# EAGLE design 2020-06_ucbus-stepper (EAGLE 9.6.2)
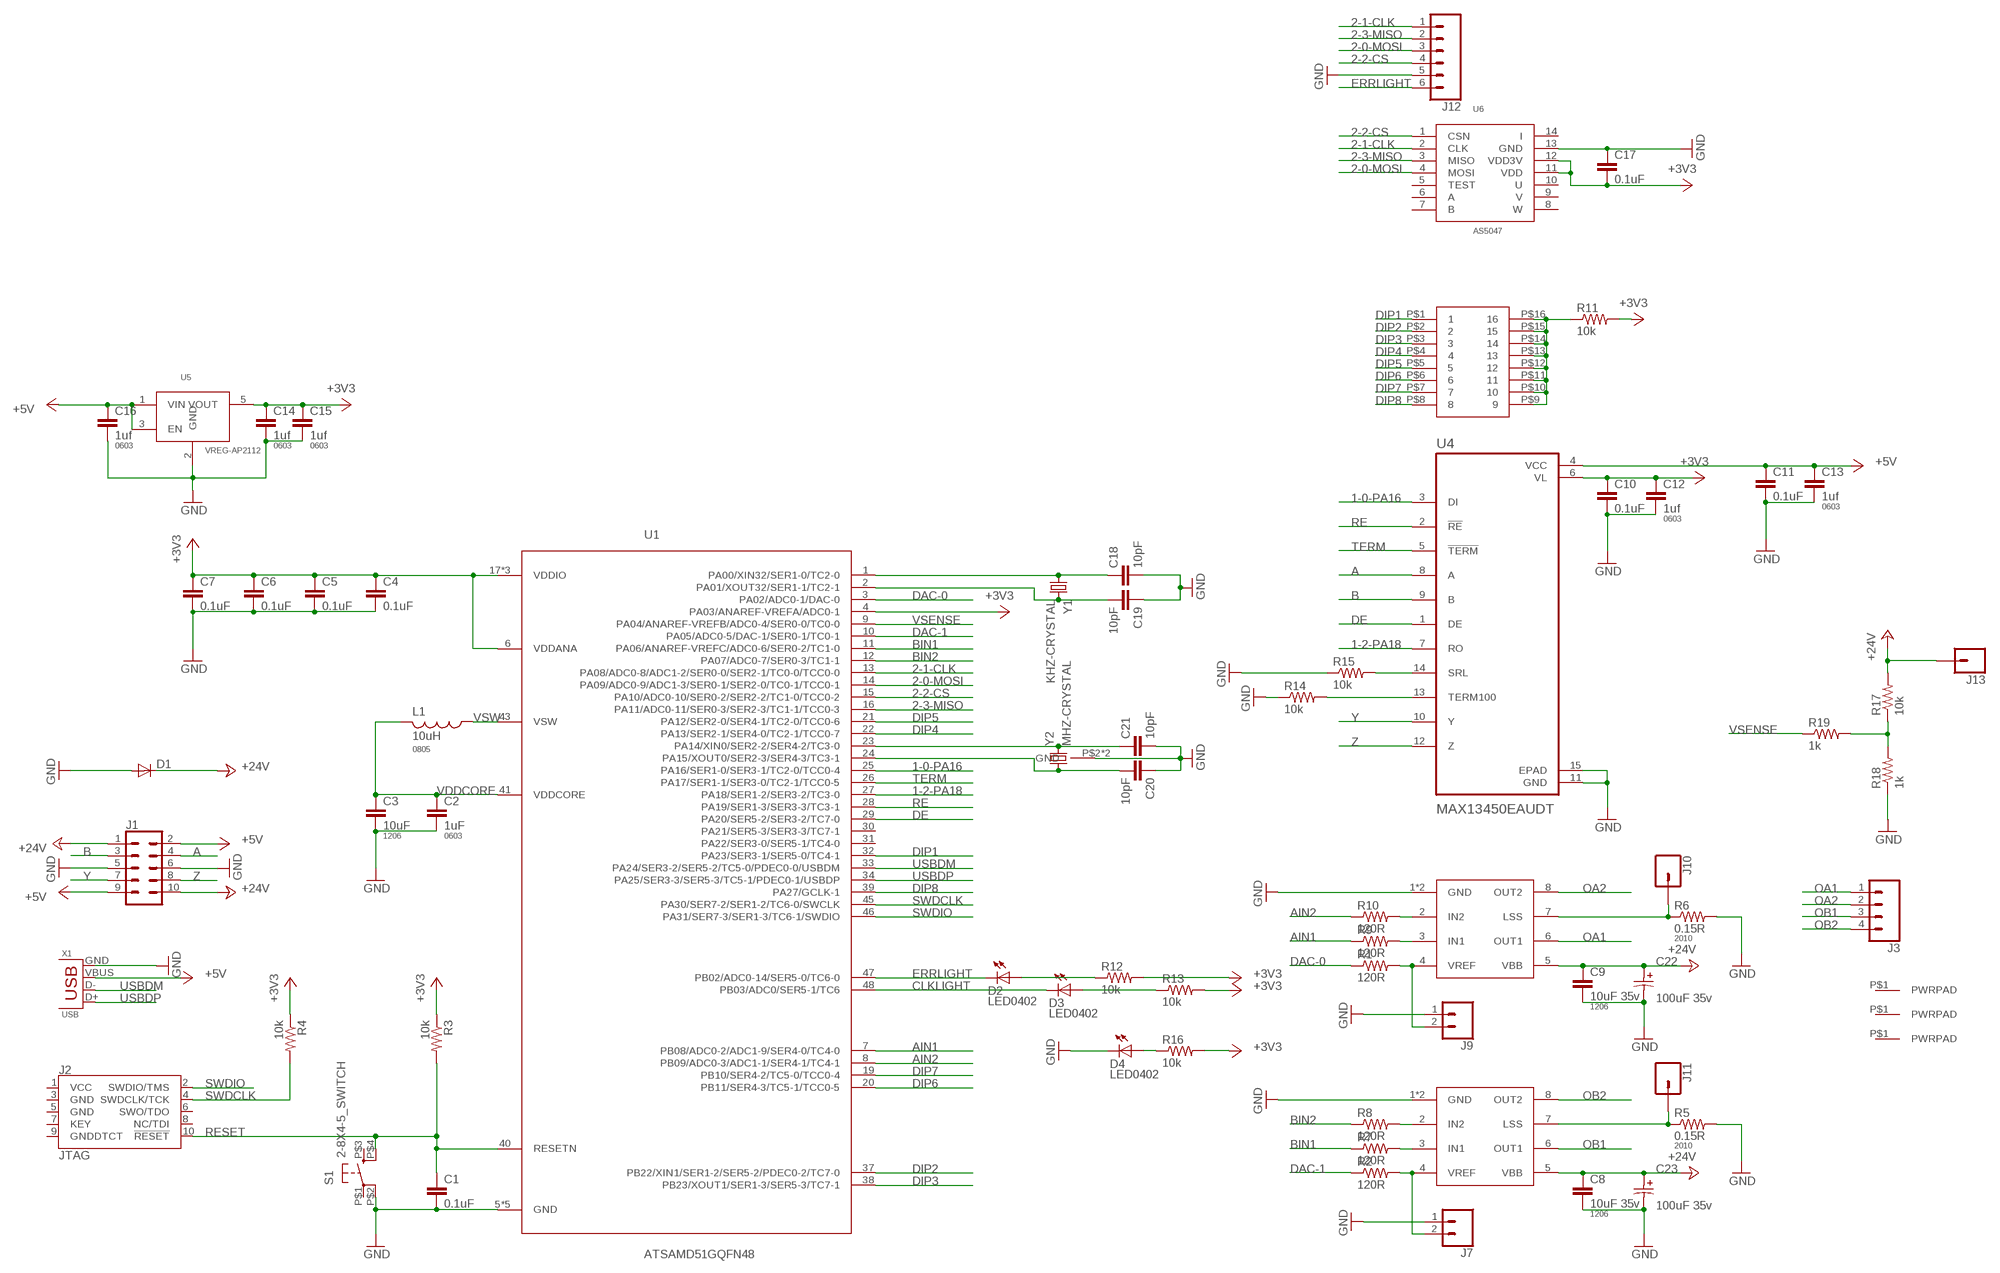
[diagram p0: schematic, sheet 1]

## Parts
C1  0.1uF  CAP0402  [0402]
C2  1uF  CAP0603-CAP  [0603-CAP]
C3  10uF  CAP1206  [1206]
C4  0.1uF  CAP0402  [0402]
C5  0.1uF  CAP0402  [0402]
C6  0.1uF  CAP0402  [0402]
C7  0.1uF  CAP0402  [0402]
C8  10uF 35v  CAP1206  [1206]
C9  10uF 35v  CAP1206  [1206]
C10  0.1uF  CAP0402  [0402]
C11  0.1uF  CAP0402  [0402]
C12  1uf  CAP0603-CAP  [0603-CAP]
C13  1uf  CAP0603-CAP  [0603-CAP]
C14  1uf  CAP0603-CAP  [0603-CAP]
C15  1uf  CAP0603-CAP  [0603-CAP]
C16  1uf  CAP0603-CAP  [0603-CAP]
C17  0.1uF  CAP0402  [0402]
C18  10pF  CAP0402  [0402]
C19  10pF  CAP0402  [0402]
C20  10pF  CAP0402  [0402]
C21  10pF  CAP0402  [0402]
C22  100uF 35v  CAP-POLCAP_POL_SMD6.6X6.6  [SMD-ELEC-CAP]
C23  100uF 35v  CAP-POLCAP_POL_SMD6.6X6.6  [SMD-ELEC-CAP]
D1  DIODESMA403D  [SMA-403D]
D2  LED0402  [0402-D]
D3  LED0402  [0402-D]
D4  LED0402  [0402-D]
J1  CONN_05X2SHD_SMD  [2X5-SHROUDED_SMD]
J2  JTAG  CORTEX_JTAG_DEBUG_SMD  [2X5-SMD-1.27MM]
J3  CONN_04SCREW_LOCK  [SCREWTERMINAL-3.5MM-4_LOCK]
J4  PWRPADM3-SKINNY  [PWRPAD_3-25MM-SKINNY]
J5  PWRPADM3-SKINNY  [PWRPAD_3-25MM-SKINNY]
J6  PWRPADM3-SKINNY  [PWRPAD_3-25MM-SKINNY]
J7  CONN_02LOCK  [1X02_LOCK]
J8  DIPSWITCH-8  [DIPSWITCH-8]
J9  CONN_02LOCK  [1X02_LOCK]
J10  CONN_01PTH_NO_SILK_YES_STOP  [1X01_NO_SILK]
J11  CONN_01PTH_NO_SILK_YES_STOP  [1X01_NO_SILK]
J12  CONN_06SMD-FEMALE-V2  [1X06-SMD-FEMALE]
J13  CONN_01PTH_NO_SILK_YES_STOP  [1X01_NO_SILK]
L1  10uH  INDUCTOR-0805  [0805]
R1  120R  RESISTOR0402  [0402]
R2  120R  RESISTOR0402  [0402]
R3  10k  RESISTOR0402  [0402]
R4  10k  RESISTOR0402  [0402]
R5  0.15R  RESISTOR2010  [R2010]
R6  0.15R  RESISTOR2010  [R2010]
R7  120R  RESISTOR0402  [0402]
R8  120R  RESISTOR0402  [0402]
R9  120R  RESISTOR0402  [0402]
R10  120R  RESISTOR0402  [0402]
R11  10k  RESISTOR0402  [0402]
R12  10k  RESISTOR0402  [0402]
R13  10k  RESISTOR0402  [0402]
R14  10k  RESISTOR0402  [0402]
R15  10k  RESISTOR0402  [0402]
R16  10k  RESISTOR0402  [0402]
R17  10k  RESISTOR0402  [0402]
R18  1k  RESISTOR0402  [0402]
R19  1k  RESISTOR0402  [0402]
S1  2-8X4-5_SWITCH  [TACT-SWITCH-KMR6]
U1  ATSAMD51GQFN48  [QFN-48-7X7MM]
U2  A4950  [SOIC8_PAD]
U3  A4950  [SOIC8_PAD]
U4  MAX13450EAUDT  [SOP65P637X110-14N]
U5  VREG-AP2112  [SOT23-5]
U6  AS5047  [TSSOP14]
X1  USB  [USB_MICRO_609-4613-1-ND]
Y1  KHZ-CRYSTAL  [2-SMD-3.2X1.5MM]
Y2  MHZ-CRYSTAL  [4-SMD-3.2X2.5]

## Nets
1-0-PA16: U1.25(PA16/SER1-0/SER3-1/TC2-0/TCC0-4) U4.3(DI)
1-2-PA18: U1.27(PA18/SER1-2/SER3-2/TC3-0) U4.7(RO)
2-0-MOSI: J12.3 U1.14(PA09/ADC0-9/ADC1-3/SER0-1/SER2-0/TC0-1/TCC0-1) U6.4(MOSI)
2-1-CLK: J12.1 U1.13(PA08/ADC0-8/ADC1-2/SER0-0/SER2-1/TC0-0/TCC0-0) U6.2(CLK)
2-2-CS: J12.4 U1.15(PA10/ADC0-10/SER0-2/SER2-2/TC1-0/TCC0-2) U6.1(CSN)
2-3-MISO: J12.2 U1.16(PA11/ADC0-11/SER0-3/SER2-3/TC1-1/TCC0-3) U6.3(MISO)
+3V3: C4.1 C5.1 C6.1 C7.1 C10.1 C12.1 C14.1 C15.1 C17.2 R3.1 R4.1 R11.2 R12.2 R13.2 R16.2 U1.4(PA03/ANAREF-VREFA/ADC0-1) U1.6(VDDANA) U1.17(VDDIO) U1.36(VDDIO) U1.44(VDDIO) U4.6(VL) U5.5(VOUT) U6.11(VDD) U6.12(VDD3V)
+5V: C11.1 C13.1 C16.1 J1.2 J1.9 U4.4(VCC) U5.1(VIN) U5.3(EN) X1.VBUS
+24V: C8.1 C9.1 C22.A C23.A D1.P$1(C) J1.1 J1.10 J13.1 R17.2 U2.5(VBB) U3.5(VBB)
A: J1.4 U4.8(A)
AIN1: R9.1 U1.7(PB08/ADC0-2/ADC1-9/SER4-0/TC4-0)
AIN2: R10.1 U1.8(PB09/ADC0-3/ADC1-1/SER4-1/TC4-1)
B: J1.3 U4.9(B)
BIN1: R7.1 U1.11(PA06/ANAREF-VREFC/ADC0-6/SER0-2/TC1-0)
BIN2: R8.1 U1.12(PA07/ADC0-7/SER0-3/TC1-1)
CLKLIGHT: D3.1(C) U1.48(PB03/ADC0/SER5-1/TC6)
DAC-0: R1.1 U1.3(PA02/ADC0-1/DAC-0)
DAC-1: R2.1 U1.10(PA05/ADC0-5/DAC-1/SER0-1/TC0-1)
DE: U1.29(PA20/SER5-2/SER3-2/TC7-0) U4.1(DE)
DIP1: J8.P$1 U1.32(PA23/SER3-1/SER5-0/TC4-1)
DIP2: J8.P$2 U1.37(PB22/XIN1/SER1-2/SER5-2/PDEC0-2/TC7-0)
DIP3: J8.P$3 U1.38(PB23/XOUT1/SER1-3/SER5-3/TC7-1)
DIP4: J8.P$4 U1.22(PA13/SER2-1/SER4-0/TC2-1/TCC0-7)
DIP5: J8.P$5 U1.21(PA12/SER2-0/SER4-1/TC2-0/TCC0-6)
DIP6: J8.P$6 U1.20(PB11/SER4-3/TC5-1/TCC0-5)
DIP7: J8.P$7 U1.19(PB10/SER4-2/TC5-0/TCC0-4)
DIP8: J8.P$8 U1.39(PA27/GCLK-1)
ERRLIGHT: D2.1(C) J12.6 U1.47(PB02/ADC0-14/SER5-0/TC6-0)
GND: C1.2 C2.2 C3.2 C4.2 C5.2 C6.2 C7.2 C8.2 C9.2 C10.2 C11.2 C12.2 C13.2 C14.2 C15.2 C16.2 C17.1 C18.2 C19.1 C20.1 C21.2 C22.C C23.C D1.P$2(A) D4.1(C) J1.5 J1.6 J7.1 J9.1 J12.5 R5.2 R6.2 R14.1 R15.1 R18.1 S1.P$2(P1) U1.5(GND) U1.18(GND) U1.35(GND) U1.42(GND) U1.P$1(GND) U2.1(GND) U2.P$1(GND) U3.1(GND) U3.P$1(GND) U4.11(GND) U4.15(EPAD) U5.2(GND) U6.13(GND) X1.GND Y2.P$2(GND) Y2.P$4(GND)
N$1: R9.2 U3.3(IN1)
N$2: J7.2 R2.2 U2.4(VREF)
N$3: J9.2 R1.2 U3.4(VREF)
N$4: R10.2 U3.2(IN2)
N$5: J10.1 R6.1 U3.7(LSS)
N$6: J11.1 R5.1 U2.7(LSS)
N$7: R8.2 U2.2(IN2)
N$8: R7.2 U2.3(IN1)
N$9: J8.P$9 J8.P$10 J8.P$11 J8.P$12 J8.P$13 J8.P$14 J8.P$15 J8.P$16 R11.1
N$10: C18.1 U1.1(PA00/XIN32/SER1-0/TC2-0) Y1.P$1
N$11: C19.2 U1.2(PA01/XOUT32/SER1-1/TC2-1) Y1.P$2
N$12: C21.1 U1.23(PA14/XIN0/SER2-2/SER4-2/TC3-0) Y2.P$3
N$13: C20.2 U1.24(PA15/XOUT0/SER2-3/SER4-3/TC3-1) Y2.P$1
N$14: D3.2(A) R13.1
N$15: D2.2(A) R12.1
N$16: D4.2(A) R16.1
N$17: R17.1 R18.2 R19.2
N$18: R14.2 U4.13(TERM100)
N$19: R15.2 U4.14(SRL)
OA1: J3.1 U3.6(OUT1)
OA2: J3.2 U3.8(OUT2)
OB1: J3.3 U2.6(OUT1)
OB2: J3.4 U2.8(OUT2)
RE: U1.28(PA19/SER1-3/SER3-3/TC3-1) U4.2(!RE)
RESET: C1.1 J2.10(!RESET) R3.2 S1.P$4(S1) U1.40(RESETN)
SWDCLK: J2.4(SWDCLK/TCK) R4.2 U1.45(PA30/SER7-2/SER1-2/TC6-0/SWCLK)
SWDIO: J2.2(SWDIO/TMS) U1.46(PA31/SER7-3/SER1-3/TC6-1/SWDIO)
TERM: U1.26(PA17/SER1-1/SER3-0/TC2-1/TCC0-5) U4.5(!TERM)
USBDM: U1.33(PA24/SER3-2/SER5-2/TC5-0/PDEC0-0/USBDM) X1.D-
USBDP: U1.34(PA25/SER3-3/SER5-3/TC5-1/PDEC0-1/USBDP) X1.D+
VDDCORE: C2.1 C3.1 L1.2 U1.41(VDDCORE)
VSENSE: R19.1 U1.9(PA04/ANAREF-VREFB/ADC0-4/SER0-0/TC0-0)
VSW: L1.1 U1.43(VSW)
Y: J1.7 U4.10(Y)
Z: J1.8 U4.12(Z)
Unconnected: J2.1(VCC) J2.3(GND) J2.5(GND) J2.6(SWO/TDO) J2.7(KEY) J2.8(NC/TDI) J2.9(GNDDTCT) J4.P$1(PWRPAD) J5.P$1(PWRPAD) J6.P$1(PWRPAD) S1.P$1(P) S1.P$3(S) U1.30(PA21/SER5-3/SER3-3/TC7-1) U1.31(PA22/SER3-0/SER5-1/TC4-0) U6.5(TEST) U6.6(A) U6.7(B) U6.8(W) U6.9(V) U6.10(U) U6.14(I)

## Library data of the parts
C1 C4-C7 C10 C11 C17-C21 = passives:CAP: Capacitor
C2 C12-C16 = passives:CAP: Capacitor; PACKAGE: 0603
C3 C8 C9 = passives:CAP: Capacitor; PACKAGE: 1206
C22 C23 = passives:CAP-POL
D1 = passives:DIODE: DIODE
D2-D4 = lights:LED: LED
J1 = SparkFun-Connectors:CONN_05X2: Multi connection point. Often used as Generic Header-pin footprint for 0.1 inch spaced/style header connections For AVR SPI programming port, see special device with nice symbol: "AVR_SPI_PROG_5x2.dev" You can populate with any combo of single row headers, but if you'd like an exact match, check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; PROD_ID: CONN-09508
J2 = SparkFun-Connectors:CORTEX_JTAG_DEBUG: Cortex Debug Connector - 10 pin Supports JTAG debug, Serial Wire debug, and Serial Wire Viewer. PTH and SMD connector options available. General Connector Information Products: PTH Connector -via Digi-Key SparkFun PSoc SparkFun T; PROD_ID: CONN-14503
J3 = SparkFun-Connectors:CONN_04: Multi connection point. Often used as Generic Header-pin footprint for 0.1 inch spaced/style header connections On any of the 0.1 inch spaced packages, you can populate with these: Break Away Headers - Straight (PRT-00116) Break Away Male Headers - Right Angle (PRT-00553) Female Headers (PRT-00115)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
J4-J6 = connector:PWRPAD
J7 J9 = SparkFun-Connectors:CONN_02: Multi connection point. Often used as Generic Header-pin footprint for 0.1 inch spaced/style header connections
J8 = passives:DIPSWITCH-8
J10 J11 J13 = SparkFun-Connectors:CONN_01: Single connection point. Often used as Generic Header-pin footprint for 0.1 inch spaced/style header connections
J12 = SparkFun-Connectors:CONN_06: Multi connection point. Often used as Generic Header-pin footprint for 0.1 inch spaced/style header connections On any of the 0.1 inch spaced packages, you can populate with these: Break Away Headers - Straight (PRT-00116) Break Away Male Headers - Right Angle (PRT-00553) Female Headers (PRT-00115)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; PROD_ID: CONN-09668
L1 = passives:INDUCTOR; PACKAGE: 0805
R1-R4 R7-R19 = passives:RESISTOR: Resistor
R5 R6 = passives:RESISTOR: Resistor; PACKAGE: 2010
S1 = passives:2-8X4-5_SWITCH
U1 = microcontrollers:ATSAMD51G
U2 U3 = power:A4950
U4 = comm:MAX13450EAUDT; DESCRIPTION: 1/1 Transceiver Full RS422, RS485 14-TSSOP-EP; DIGI-KEY_PART_NUMBER: MAX13450EAUD+T-ND; DIGIKEY-PURCHASE-URL: https://snapeda.com/shop?store=DigiKey&id=694117; MF: Maxim Integrated; MP: MAX13450EAUD+; PACKAGE: TSSOP-14 Maxim
U5 = power:VREG-AP2112
U6 = sensor:AS5047
X1 = connector:USB: SMD micro USB connector as found in the fablab inventory. Three footprint variants included: original, as described by manufacturer's datasheet for milling with the 1/100" bit for milling with the 1/64" bit Made by Zaerc.
Y1 = passives:KHZ-CRYSTAL
Y2 = passives:MHZ-CRYSTAL

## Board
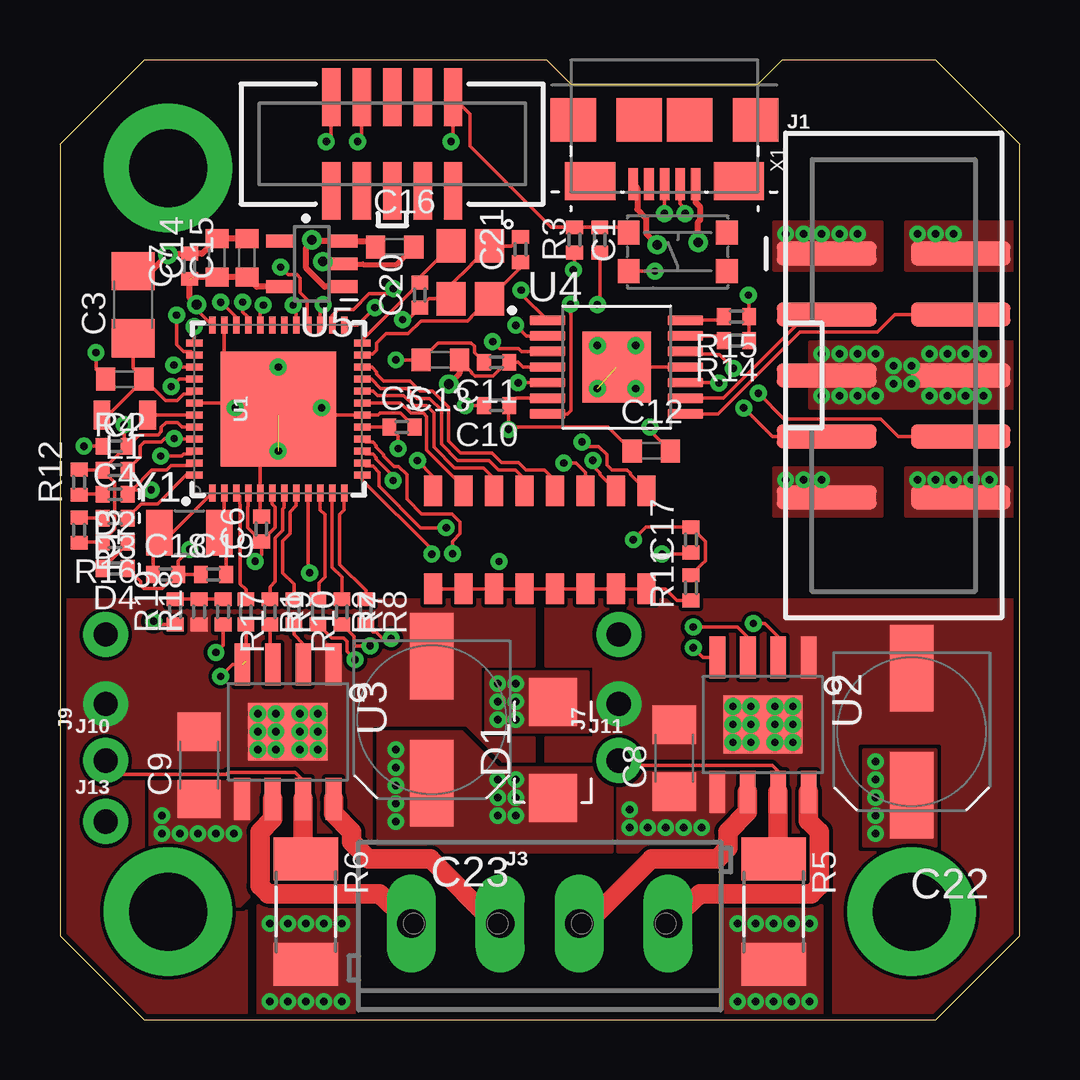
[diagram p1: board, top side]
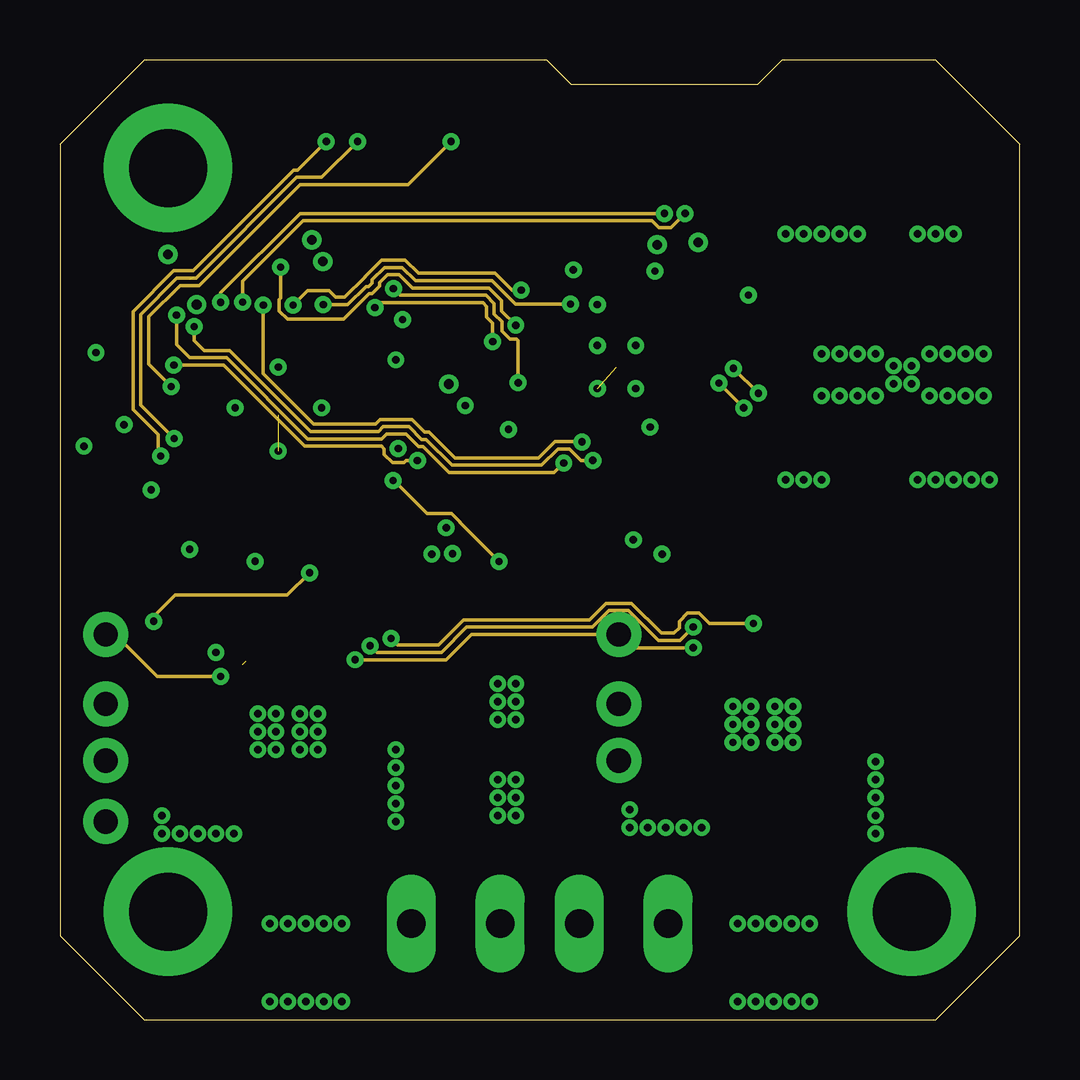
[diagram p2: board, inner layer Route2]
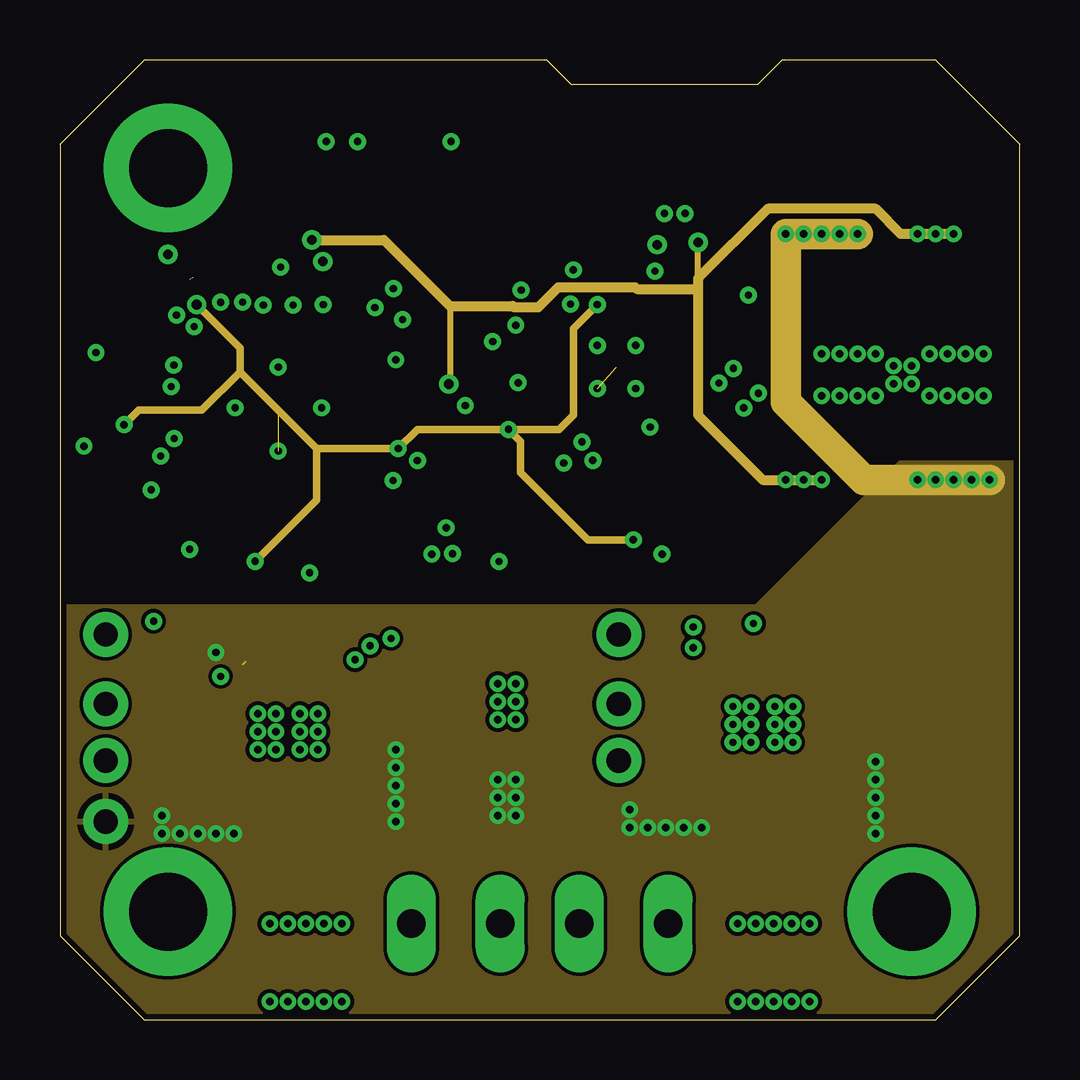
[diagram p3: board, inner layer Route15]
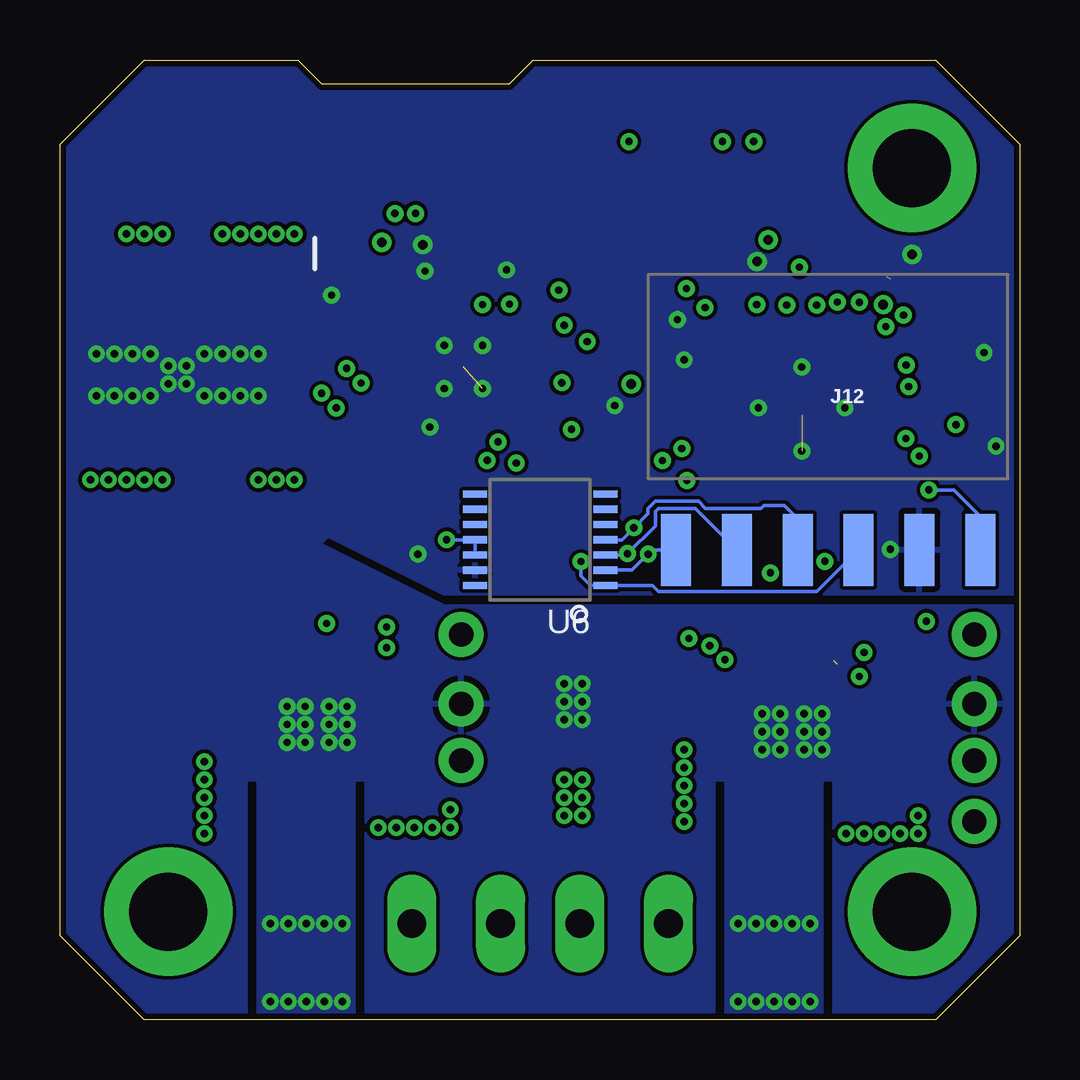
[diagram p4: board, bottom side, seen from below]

Size 40 x 40 mm. Coordinates in mm from the lower left corner, seen from the top.
Outline: 3.5,0 36.5,0 40,3.5 40,36.5 36.5,40 30.1,40 29.1,39 21.3,39 20.3,40 3.5,40 0,36.5 0,3.5 3.5,0
Copper layers (1+2*15+16): Top 0.035mm / dielectric 1.5mm / Route2 0.035mm / dielectric 0.15mm / Route15 0.035mm / dielectric 0.2mm / Bottom 0.035mm
Design rules "default *": minimum track width 6mil, minimum drill 10mil, track to track 6mil, track to pad 6mil, pad to pad 6mil, via to via 6mil, smd to smd 0mil, copper to edge 10mil, drill to drill 6mil, minimum pad ring 10mil, minimum via ring 8mil, stop-mask expansion 4mil, vias tented up to drill 35mil, thermal gap 10mil

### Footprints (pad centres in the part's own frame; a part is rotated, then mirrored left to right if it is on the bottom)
0402 = smd 0.575 x 0.7: 1 -0.525,0; 2 0.525,0
0603-CAP = smd 0.8 x 0.95: 1 -0.8,0; 2 0.8,0
1206 = smd 1.6 x 1.8: 1 -1.4,0; 2 1.4,0
SMD-ELEC-CAP = smd 1.8 x 3.6: A 0,2.65; C 0,-2.65
SMA-403D = smd 2 x 2: P$1 -2,0; P$2 2,0
0402-D = smd 0.575 x 0.7: 1 -0.525,0; 2 0.525,0
2X5-SHROUDED_SMD = smd 4.15 x 1: 1 -2.794,5.08; 2 2.794,5.08; 3 -2.794,2.54; 4 2.794,2.54; 5 -2.794,0; 6 2.794,0; 7 -2.794,-2.54; 8 2.794,-2.54; 9 -2.794,-5.08; 10 2.794,-5.08
2X5-SMD-1.27MM = smd 0.76 x 2.4: 1 2.54,1.95; 2 2.54,-1.95; 3 1.27,1.95; 4 1.27,-1.95; 5 0,1.95; 6 0,-1.95; 7 -1.27,1.95; 8 -1.27,-1.95; 9 -2.54,1.95; 10 -2.54,-1.95
SCREWTERMINAL-3.5MM-4_LOCK = drill 1.2 pad 2.032 long: 1 -0.1,0; 2 3.6,0; 3 6.9,0; 4 10.6,0
PWRPAD_3-25MM-SKINNY = drill 3.25 pad 5.35: P$1 0,0
1X02_LOCK = drill 1.016 pad 1.88: 1 -0.178,0; 2 2.718,0
DIPSWITCH-8 = smd 0.737 x 1.27: P$1 -4.445,-2.045; P$2 -3.175,-2.045; P$3 -1.905,-2.045; P$4 -0.635,-2.045; P$5 0.635,-2.045; P$6 1.905,-2.045; P$7 3.175,-2.045; P$8 4.445,-2.045; P$9 4.445,2.045; P$10 3.175,2.045; P$11 1.905,2.045; P$12 0.635,2.045; P$13 -0.635,2.045; P$14 -1.905,2.045; P$15 -3.175,2.045; P$16 -4.445,2.045
1X01_NO_SILK = drill 1.016 pad 1.88: 1 0,0
1X06-SMD-FEMALE = smd 1.25 x 3: 1 6.35,3.425; 2 3.81,3.425; 3 1.27,3.425; 4 -1.27,3.425; 5 -3.81,3.425; 6 -6.35,3.425
0805 = smd 0.7 x 1.2: 1 -0.95,0; 2 0.95,0
R2010 = smd 1.8 x 2.7: 1 -2.2,0; 2 2.2,0
TACT-SWITCH-KMR6 = smd 0.9 x 1: P$1 -2.05,0.8; P$2 2.05,0.8; P$3 -2.05,-0.8; P$4 2.05,-0.8
QFN-48-7X7MM = smd 0.7 x 0.275: 1 -3.5,2.75; 2 -3.5,2.25; 3 -3.5,1.75; 4 -3.5,1.25; 5 -3.5,0.75; 6 -3.5,0.25; 7 -3.5,-0.25; 8 -3.5,-0.75; 9 -3.5,-1.25; 10 -3.5,-1.75; 11 -3.5,-2.25; 12 -3.5,-2.75; 25 3.5,-2.75; 26 3.5,-2.25; 27 3.5,-1.75; 28 3.5,-1.25; 29 3.5,-0.75; 30 3.5,-0.25; 31 3.5,0.25; 32 3.5,0.75; 33 3.5,1.25; 34 3.5,1.75; 35 3.5,2.25; 36 3.5,2.75 | smd 0.275 x 0.7: 13 -2.75,-3.5; 14 -2.25,-3.5; 15 -1.75,-3.5; 16 -1.25,-3.5; 17 -0.75,-3.5; 18 -0.25,-3.5; 19 0.25,-3.5; 20 0.75,-3.5; 21 1.25,-3.5; 22 1.75,-3.5; 23 2.25,-3.5; 24 2.75,-3.5; 37 2.75,3.5; 38 2.25,3.5; 39 1.75,3.5; 40 1.25,3.5; 41 0.75,3.5; 42 0.25,3.5; 43 -0.25,3.5; 44 -0.75,3.5; 45 -1.25,3.5; 46 -1.75,3.5; 47 -2.25,3.5; 48 -2.75,3.5 | smd 4.8 x 4.8: P$1 0,0
SOIC8_PAD = smd 1.75 x 0.65: 1 -2.8,1.905; 2 -2.8,0.645; 3 -2.8,-0.625; 4 -2.8,-1.895; 5 2.8,-1.905; 6 2.8,-0.635; 7 2.8,0.635; 8 2.8,1.905 | smd 2.41 x 3.3: P$1 0,0
SOP65P637X110-14N = smd 1.48 x 0.41: 1 -2.875,1.95; 2 -2.875,1.3; 3 -2.875,0.65; 4 -2.875,0; 5 -2.875,-0.65; 6 -2.875,-1.3; 7 -2.875,-1.95; 8 2.875,-1.95; 9 2.875,-1.3; 10 2.875,-0.65; 11 2.875,0; 12 2.875,0.65; 13 2.875,1.3; 14 2.875,1.95 | smd 2.85 x 2.95: 15 0,0
SOT23-5 = smd 0.533 x 1.194: 1 -0.95,-1.306; 2 0,-1.306; 3 0.95,-1.306; 4 0.95,1.306; 5 -0.95,1.306
TSSOP14 = smd 0.305 x 0.991: 1 -1.905,-2.718; 2 -1.27,-2.718; 3 -0.635,-2.718; 4 0,-2.718; 5 0.635,-2.718; 6 1.27,-2.718; 7 1.905,-2.718; 8 1.905,2.718; 9 1.27,2.718; 10 0.635,2.718; 11 0,2.718; 12 -0.635,2.718; 13 -1.27,2.718; 14 -1.905,2.718
USB_MICRO_609-4613-1-ND = smd 0.4 x 1.35: D+ 0,2.675; D- -0.65,2.675; GND 1.3,2.675; ID 0.65,2.675; VBUS -1.3,2.675 | smd 1.9 x 1.8: HD0 -3.8,0; HD1 -1.05,0; HD2 1.05,0; HD3 3.8,0 | smd 2.1 x 1.6: HD4 -3.1,2.55; HD5 3.1,2.55
2-SMD-3.2X1.5MM = smd 1.1 x 1.9: P$1 -1.25,0; P$2 1.25,0
4-SMD-3.2X2.5 = smd 1.4 x 1.2: P$1 -1.1,-0.8; P$2 1.1,-0.8; P$3 1.1,0.8; P$4 -1.1,0.8

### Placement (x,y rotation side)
C1  21.45,32.5 270 top
C2  2.7,26.7 180 top
C3  3.05,29.8 90 top
C4  2.3,23.9 180 top
C5  14.25,24.7 0 top
C6  8.4,20.45 90 top
C7  5.4,31.4 90 top
C8  25.6,10.9 90 top
C9  5.8,10.6 90 top
C10  18.2,25.6 180 top
C11  18.2,27.4 180 top
C12  24.65,23.7 0 top
C13  15.85,27.5 180 top
C14  6.55,31.75 90 top
C15  7.8,31.75 90 top
C16  13.95,32.2 0 top
C17  26.3,20 90 top
C18  4.4,18.55 0 top
C19  6.4,18.55 0 top
C20  15,30.2 90 top
C21  19.2,32.1 90 top
C22  35.5,12 180 top
C23  15.5,12.5 180 top
D1  20.55,11.25 90 top
D2  2.3,21.9 180 top
D3  2.3,20.9 180 top
D4  2.3,18.8 180 top
J1  34.75,26.85 0 top
J2  13.85,36.5 180 top
J3  14.75,4 0 top
J4  35.5,4.5 0 top
J5  4.5,35.5 0 top
J6  4.5,4.5 0 top
J7  23.3,13.34 90 top
J8  20,20 180 top
J9  1.91,13.34 90 top
J10  1.91,10.79 0 top
J11  23.3,10.79 0 top
J12  8,23 180 bottom
J13  1.91,8.26 0 top
L1  2.7,25.2 180 top
R1  7.75,17 270 top
R2  10.75,17 270 top
R3  22.5,32.5 90 top
R4  2.3,22.9 0 top
R5  29.75,4.5 270 top
R6  10.25,4.5 270 top
R7  11.75,17 270 top
R8  12.75,17 270 top
R9  8.75,17 270 top
R10  9.75,17 270 top
R11  26.3,18 90 top
R12  0.8,22.4 90 top
R13  0.8,20.4 270 top
R14  28.2,28.3 180 top
R15  28.2,29.3 180 top
R16  2.3,19.9 180 top
R17  6.8,17 270 top
R18  5.8,17 90 top
R19  4.8,17 90 top
S1  25.75,32 180 top
U1  9.1,25.45 90 top
U2  29.3,12.3 270 top
U3  9.5,12 270 top
U4  23.2,27.2 0 top
U5  10.5,31.5 90 top
U6  20,20 90 bottom
X1  25.2,37.5 180 top
Y1  5.4,20.3 0 top
Y2  17.1,31.15 270 top

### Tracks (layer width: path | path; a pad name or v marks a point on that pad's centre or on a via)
1-0-PA16  (via drill 0.3)
  Top 0.152: U4.3 19.24,27.85 19.11,27.98 18.32,27.98 v18.04,28.26 | v13.13,29.67 12.4,28.95 U1.25
  Route2 0.152: v18.04,28.26 18.04,29.04 17.79,29.29 17.79,29.72 17.63,29.89 13.34,29.89 v13.13,29.67
1-2-PA18  (via drill 0.3)
  Top 0.152: U1.27 10.85,29.67 v10.98,29.8 | v21.29,29.82 21.29,29.43 21.29,29.42 21.29,25.39 21.15,25.25 U4.7
  Route2 0.152: v10.98,29.8 12,29.8 12.76,30.56 12.87,30.56 13.01,30.7 13.01,30.84 13.53,31.35 14.27,31.35 14.82,30.8 18.01,30.8 18.99,29.82 v21.29,29.82
2-0-MOSI  (via drill 0.3)
  Top 0.152: U1.14 12.73,23.07 13.04,23.07 13.3,22.81 13.3,22.23 15.03,20.5 v16.1,20.5
  Bottom 0.152: U6.4 16.6,20 v16.1,20.5 15.51,21.09 15.51,21.3 15.2,21.61 13.41,21.61 13.11,21.3 10.8,21.3 10.68,21.42 9.82,21.42 9.27,20.87 J12.3
2-1-CLK  (via drill 0.3)
  Top 0.152: U1.13 12.6,22.5 15.5,19.6 v15.5,19.4
  Bottom 0.152: U6.2 16.17,18.73 v15.5,19.4 15.32,19.57 J12.1
2-2-CS  (via drill 0.3)
  Top 0.152: v13.88,22.47 13.88,22.67 13.87,22.67 13.18,23.36 13.18,23.43 13.04,23.57 12.73,23.57 U1.15
  Route2 0.152: v18.3,19.1 16.68,20.71 16.68,20.74 16.32,21.1 15.3,21.1 13.93,22.47 v13.88,22.47
  Bottom 0.152: v18.3,19.1 18.3,18.5 17.9,18.1 U6.1 15.32,18.09 15.07,17.85 8.46,17.85 J12.4
2-3-MISO  (via drill 0.3)
  Top 0.152: v16.36,19.42 16.36,19.94 16.68,20.26 16.68,20.74 16.34,21.08 15.08,21.08 14.46,21.7 14.46,22.71 14.12,23.05 13.92,23.05 13.48,23.49 13.48,23.56 13.18,23.86 13.18,23.93 13.04,24.07 12.73,24.07 U1.16
  Bottom 0.152: U6.3 16.41,19.36 v16.36,19.42 15.2,20.57 15.2,21.17 15.07,21.3 13.54,21.3 J12.2
+3V3  (via drill 0.3, 0.4)  (1 unrouted)
  Top 0.152: U1.4 7.85,21.39 7.82,21.36 7.82,20.5 C6.1 | U1.6 8.85,21.49 8.98,21.36 8.98,20.5 C6.1 | 5.4,30.7 C7.1 | U1.44 5.1,24.7 4.91,24.89 4.42,24.89 4.23,24.7 4.23,24.5 4.09,24.37 3.3,24.37 C4.1 | R4.1 0.82,22.9 R12.2 | R4.1 2.77,23.9 C4.1 | v23.9,20 24.43,20.52 C17.2 26.9,19.93 26.9,19.11 26.75,18.96 26.73,18.96 R11.2 | U1.17 C5.1 14.1,24.32 v14.1,23.8 | U4.6 19.02,25.9 C10.1 18.7,25.57 v18.7,24.6 18.8,24.7 22.85,24.7 C12.1 | R13.2 0.82,19.9 R16.2 1.77,19.94 2.29,20.45 2.29,22.38 R4.1 | C6.1 8.4,19.36 v8.14,19.1 | C4.1 2.67,24.06 v2.67,24.79 | U1.36 5.7,29.6 v5.7,29.8 | R3.1 22.5,29.9 v22.4,29.8
  Top 0.254: U5.5 8.2,30.55 C15.1 C14.1 5.55,30.95 | v5.7,29.8 5.4,30.1 5.4,30.7
  Route15 0.305: v5.7,29.8 7.5,28 7.5,27 | 7.5,27 10.7,23.8 | 10.7,23.8 v14.1,23.8 14.9,24.6 v18.7,24.6 | 10.7,23.8 10.7,21.66 v8.14,19.1 | v2.67,24.79 3.27,25.4 5.9,25.4 7.5,27 | v18.7,24.6 19.2,24.1 19.2,22.8 22,20 v23.9,20 | v18.7,24.6 20.8,24.6 21.4,25.2 21.4,28.8 v22.4,29.8
  Bottom 0.152: U6.12 U6.11 v23.9,20
+5V  (via drill 0.3, 0.4)
  Top 0.152: U4.4 19.3,27.2 19.1,27.4 C11.1 18.64,27.4 18.06,26.82 17.29,26.82 17.16,26.95 17.16,26.99 C13.1
  Top 0.254: C16.1 12.9,32.45 U5.3 10.55,32.45 | 10.55,32.45 v10.5,32.5 | C13.1 16.65,26.93 v16.21,26.49 | X1.VBUS 26.5,34.05 26.69,33.86 26.69,33.34 26.6,33.25 v26.6,32.4 | U5.1 11.03,30.55 10.27,31.31 10.27,32.17 10.55,32.45
  Route15 0.254: v16.21,26.49 16.25,26.54 16.25,29.75 | 26.55,30.45 26.6,30.5 v26.6,32.4
  Route15 0.406: v10.5,32.5 13.5,32.5 16.25,29.75 18.88,29.75 18.93,29.69 19.94,29.69 20.78,30.53 23.97,30.53 24.05,30.45 26.55,30.45 26.6,30.4 26.6,25.2 29.3,22.5 v30.25,22.5 v31,22.5 v31.75,22.5 | v37.25,32.75 v36.5,32.75 v35.75,32.75 35.05,32.75 34,33.8 29.5,33.8 26.6,30.9 26.6,30.5
  pour Top (no thermals): 35.25,33.25 35.25,31.25 41.25,31.25 41.25,33.25
  pour Top (no thermals): 29.75,23 29.75,21 34.25,21 34.25,23
+24V  (via drill 0.3)
  Top 0.152: R17.2 6.8,15.6 v6.5,15.3
  Route15 1.27: v33.25,32.75 v32.5,32.75 v31.75,32.75 v31,32.75 v30.25,32.75 30.25,25.75 33.5,22.5 v35.75,22.5 v36.5,22.5 v37.25,22.5 v38,22.5 v38.75,22.5
  other vias: 14,11.25 14,10.5 14,9.75 14,9 14,8.25 19,8.5 19,9.25 19,10 18.25,10 18.25,9.25 18.25,8.5 26.75,8 26,8 25.25,8 24.5,8 23.75,8 23.75,8.75 7.25,7.75 6.5,7.75 5.75,7.75 5,7.75 4.25,7.75 4.25,8.5 34,10.75 34,10 34,9.25 34,8.5 34,7.75
  pour Top (no thermals): 29.75,33.25 29.75,31.25 34.25,31.25 34.25,33.25
  pour Top (no thermals): 35.25,23 35.25,21 40.25,21 40.25,23
  pour Route15: 41.5,17.5 41.5,-2.25 -1.5,-2.25 -1.5,17.25 29,17.25 35,23.25 41.5,23.25
  pour Top (no thermals): 13.25,12 16.75,12 18.25,10.5 23,10.5 23,7 13.25,7
  pour Top (no thermals): 23.25,10.5 28.25,10.5 28.25,8.5 26.75,7 23.25,7
  pour Top (no thermals): 33.5,11.25 36.5,11.25 36.5,7.25 33.5,7.25
  pour Top (no thermals): 4.5,10.25 8.75,10.25 8.75,8.25 8.25,7.75 8.25,6.75 8.25,5.5 7.5,4.75 7,4.75 5.75,4.75 3.75,6.75 3.75,9.75 3.75,10.25
A
  Top 0.152: J1.4 34.79,29.39 34.06,28.66 30.84,28.66 27.43,25.25 U4.8
AIN1
  Top 0.152: U1.7 9.35,21.35 9.28,21.28 9.28,20.38 8.98,20.07 8.98,18.25 8.75,18.02 R9.1
AIN2
  Top 0.152: U1.8 9.85,21.42 9.59,21.16 9.59,20.25 9.28,19.95 9.28,18.62 9.75,18.15 R10.1
B
  Top 0.152: U4.9 27.65,25.9 31.14,29.39 J1.3
BIN1
  Top 0.152: U1.11 11.35,18.85 11.75,18.45 R7.1
BIN2
  Top 0.152: U1.12 11.85,21.25 11.65,21.05 11.65,18.98 12.75,17.88 R8.1
CLKLIGHT
  Top 0.152: D3.1 2.83,20.94 3.38,21.5 4.07,21.5 5.27,22.7 U1.48
DAC-0
  Top 0.152: U1.3 7.48,21.82 7.48,21.5 7.52,21.47 7.52,18.16 7.75,17.93 R1.1
DAC-1
  Top 0.152: R2.1 10.85,17.62 10.8,17.68 10.8,18.2 11.04,18.45 11.04,21.05 10.85,21.25 U1.10
DE  (via drill 0.3)
  Top 0.152: U4.1 19.23,30.25 v19.23,30.4 | v9.72,29.78 9.85,29.65 U1.29
  Route2 0.152: v19.23,30.4 18.84,30.4 18.13,31.11 14.95,31.11 14.39,31.66 13.41,31.66 12.71,30.96 12.71,30.94 11.87,30.11 11.49,30.11 11.22,30.38 10.33,30.38 v9.72,29.78
DIP1  (via drill 0.3)
  Top 0.152: U1.32 8.35,29.65 v8.47,29.78 | v21.77,24.08 21.95,23.89 22.45,23.89 22.79,23.55 22.79,23.11 23,22.91 23.64,22.91 23.77,22.77 23.77,22.72 J8.P$1
  Route2 0.152: v8.47,29.78 8.47,26.92 10.58,24.81 13.15,24.81 13.35,25.01 14.68,25.01 15.2,24.49 15.39,24.49 16.48,23.41 19.96,23.41 20.63,24.09 v21.76,24.09 v21.77,24.08
DIP2  (via drill 0.3)
  Top 0.152: U1.37 5.6,28.88 v5.59,28.89 | J8.P$2 22.5,22.72 22.5,22.77 22.21,23.07 v22.21,23.31
  Route2 0.152: v5.59,28.89 5.59,28.3 6,27.89 7.07,27.89 10.45,24.51 13.28,24.51 13.48,24.71 14.55,24.71 15.07,24.19 15.27,24.19 16.35,23.11 20.08,23.11 20.76,23.78 21.24,23.78 21.71,23.31 v22.21,23.31
DIP3  (via drill 0.3)
  Top 0.152: U1.38 5.47,27.83 5.16,27.83 4.86,28.13 v4.86,29.37 | v21,23.2 21.5,23.2 21.91,22.8 J8.P$3
  Route2 0.152: v4.86,29.37 4.86,28.13 5.4,27.59 6.94,27.59 10.33,24.2 13.4,24.2 13.61,24.41 14.43,24.41 14.95,23.88 15.14,23.88 16.22,22.8 20.6,22.8 v21,23.2
DIP4
  Top 0.152: U1.22 13,27.2 13.2,27 13.2,26.91 13.5,26.61 14.59,26.61 15.01,26.19 15.54,26.19 16.21,25.52 16.21,24.11 16.71,23.61 18,23.61 18.4,23.21 19.12,23.21 19.42,22.91 20.19,22.91 20.64,22.46 J8.P$4
DIP5
  Top 0.152: J8.P$5 19.3,22.11 19.3,22.6 18.99,22.91 18.27,22.91 17.88,23.3 16.58,23.3 15.9,23.98 15.9,25.4 15.41,25.89 14.88,25.89 14.46,26.31 13.37,26.31 12.98,26.7 U1.21
DIP6
  Top 0.152: U1.20 13.05,26.2 13.24,26 14.33,26 14.75,25.58 15.28,25.58 15.6,25.27 15.6,23.86 16.45,23 17.65,23 18.09,22.55 J8.P$6
DIP7
  Top 0.152: U1.19 14.21,25.7 14.63,25.28 15.16,25.28 15.29,25.14 15.29,23.73 16.75,22.27 16.75,22.12 J8.P$7
DIP8  (via drill 0.3)
  Top 0.152: v14.9,23.3 15.55,22.64 J8.P$8 | v4.75,27.28 4.83,27.2 U1.39
  Route2 0.152: v4.75,27.28 6.82,27.28 10.2,23.9 13.4,23.9 13.52,23.78 13.52,23.56 13.86,23.22 14.34,23.22 14.42,23.3 v14.9,23.3
ERRLIGHT  (via drill 0.3)
  Top 0.152: U1.47 5.5,23.1 4.64,23.1 4.44,22.9 3.83,22.9 3,22.08 | v3.8,22.08 3,22.08 | 3,22.08 D2.1
  Bottom 0.152: J12.6 1.65,20.98 2.75,22.08 v3.8,22.08
GND  (via drill 0.3, 0.4)  (2 unrouted)
  Top 0.152: C21.2 18.82,32.25 Y2.P$4 17.13,31.48 17.13,31.45 16.3,30.63 Y2.P$2 15.38,30.05 C20.1 14.51,29.18 v14.28,29.18 | C6.2 8.35,21.02 U1.5 8.35,24.7 8.93,25.27 | C17.1 26.23,19.4 v25.1,19.4 | C5.2 14.2,25.28 13.34,25.28 13.26,25.2 U1.18 11.2,25.2 v10.9,25.5 | 8.93,25.27 8.97,25.32 | 8.97,25.32 U1.P$1 | 9.1,25.2 8.97,25.32 | U1.35 6.85,27.55 6.8,27.5 6.8,27.4 8.93,25.27 | C18.2 C19.1 | C18.2 4.84,18.55 4.26,17.97 3.49,17.97 3.36,18.11 3.36,18.27 D4.1 | C18.2 4.92,19.12 v5.4,19.6 | v14,27.5 C13.2 15.75,28.2 17.14,28.2 17.28,28.07 17.28,27.8 C11.2 | C10.2 v16.9,25.6 | C12.2 24.6,24.55 v24.6,24.7 | U4.11 U4.15 | S1.P$2 v24.8,31.2 | C1.2 21.45,31.3 v21.4,31.25 | R14.1 R15.1 28.73,30.18 v28.7,30.2 | C2.2 1.5,27.1 v1.5,27.8 | C4.2 v1,23.9 | U1.42 7.1,25.7 v7.3,25.5
  Top 0.203: C16.2 14.02,31.47 12.64,31.47 12.62,31.5 U5.2 11.71,31.6 v10.95,31.6
  Top 0.254: C15.2 C14.2 5.92,31.93 C7.2 5.38,31.9 v4.5,31.9 3.8,31.2 C3.2 | X1.GND 24.07,34.65 24.07,33.77 24.43,33.42 24.43,32.77 v24.9,32.3
  other vias: 30.55,13.05 35.5,26.5 35.5,27.25 34,27.75 34,26 32.5,26 32.5,27.75 31.75,27.75 31.75,26 37,26 37,27.75 37.75,27.75 37.75,26 34.75,27.25 34.75,26.5 33.25,26 33.25,27.75 36.25,27.75 36.25,26 38.5,27.75 38.5,26 9.1,27.2 9.1,23.7 24,28.1 22.4,28.1 22.4,26.3 24,26.3 8.75,4 9.5,4 10.25,4 11,4 11.75,4 8.75,0.75 9.5,0.75 10.25,0.75 11,0.75 11.75,0.75 28.25,4 29,4 29.75,4 30.5,4 31.25,4 28.25,0.75 29,0.75 29.75,0.75 30.5,0.75 31.25,0.75 29.8,13.05 28.8,13.05 28.05,13.05 29.8,12.3 29.8,11.55 30.55,11.55 30.55,12.3 28.8,12.3 28.05,12.3 28.05,11.55 28.8,11.55 10.75,12.75 10,12.75 9,12.75 8.25,12.75 10,12 10,11.25 10.75,11.25 10.75,12 9,12 8.25,12 8.25,11.25 9,11.25 19,14 18.25,14 18.25,13.25 18.25,12.5 19,12.5 19,13.25
  pour Bottom: 40.5,40.5 40.5,-0.5 32.25,-0.5 32.25,10 31.75,10 31.75,-0.5 27.75,-0.5 27.75,10 27.25,10 27.25,-0.5 12.75,-0.5 12.75,10 12.25,10 12.25,-0.5 8.25,-0.5 8.25,10 7.75,10 7.75,-0.5 -0.5,-0.5 -0.5,17.25 24,17.25 29.17,19.83 28.83,20.17 24,17.75 -0.5,17.75 -0.5,40.5
  pour Top (no thermals): 31.25,28.25 41.25,28.25 41.25,25.5 31.25,25.5
  pour Top (rank 4, no thermals): 8.25,-1 8.25,4.75 12.25,4.75 12.25,-1
  pour Top (rank 4, no thermals): 27.75,-1.25 27.75,4.75 31.75,4.75 31.75,-1.25
  pour Top (rank 4, no thermals): -1,17.5 41,17.5 41,-1.75 32.25,-1.75 32.25,5.5 27.25,5.5 27.25,-1.75 20.25,-1.75 20.25,11.75 22.25,11.75 22.25,14.75 20.25,14.75 20.25,17.25 19.75,17.25 19.75,14.75 17.5,14.75 17.5,11.75 19.75,11.75 19.75,-1.75 12.75,-1.75 12.75,5.25 7.75,5.25 7.75,-1.75 -1,-1.75
  pour Top (no thermals): 21.75,14.5 17.75,14.5 17.75,12 22,12 22,14.5
N$1
  Top 0.152: R9.2 8.75,14.93 U3.3
N$2  (via drill 0.3)
  Top 0.152: U2.4 26.8,15.1 v26.4,15.5 | v12.3,15 11.96,15.34 11.96,15.77 11.82,15.9 11.32,15.9 R2.2
  Route2 0.152: v26.4,15.5 23.85,15.5 J7.2 17.15,16.05 16.1,15 v12.3,15
N$3  (via drill 0.3)  (1 unrouted)
  Top 0.152: R1.2 7.75,14.95 | U3.4 7.2,14.8 v6.7,14.3
  Route2 0.152: v6.7,14.3 4.06,14.3 2.31,16.05 J9.2
N$4
  Top 0.152: R10.2 9.75,16.05 10.14,15.65 U3.2
N$5
  Top 0.152: J10.1 2.47,10.23 6.93,10.23 7,10.3 9.8,10.3 10.13,9.96 U3.7
  Top 0.61: 10.13,6.82 R6.1
  Top 0.813: U3.7 10.13,6.82
N$6
  Top 0.152: U2.7 29.93,10.37 29.7,10.6 23.49,10.6 J11.1
  Top 0.813: U2.7 29.93,6.88 R5.1
N$7  (via drill 0.3)
  Top 0.152: U2.2 29.95,15.96 29.39,16.51 v28.91,16.51 | v13.8,15.89 13.45,15.89 13.17,16.16 13.06,16.16 R8.2
  Route2 0.152: v28.91,16.51 27.07,16.51 26.64,16.94 26.16,16.94 25.82,16.6 25.82,16.33 25.6,16.11 25.07,16.11 23.83,17.35 22.76,17.35 22.07,16.66 16.83,16.66 15.78,15.61 14.08,15.61 v13.8,15.89
N$8  (via drill 0.3)
  Top 0.152: R7.2 12.26,15.96 12.26,15.6 12.28,15.58 v12.93,15.58 | v26.4,16.36 28.24,16.36 28.68,15.93 U2.3
  Route2 0.152: v12.93,15.58 13.21,15.3 15.9,15.3 16.96,16.36 22.2,16.36 22.89,17.04 23.7,17.04 24.94,15.8 25.85,15.8 v26.4,16.36
N$9
  Top 0.152: J8.P$9 J8.P$10 J8.P$11 J8.P$12 J8.P$13 J8.P$14 J8.P$15 J8.P$16 25.25,17.95 25.73,17.48 R11.1
N$10
  Top 0.152: C18.1 3.88,20.02 Y1.P$1 4.7,20.3 U1.1
N$11
  Top 0.152: C19.2 6.92,20.02 Y1.P$2 6.85,20.5 U1.2
N$12
  Top 0.152: U1.23 12.63,27.73 13.03,27.73 13.2,27.9 13.2,28.2 13.6,28.6 14.52,28.6 15.04,29.12 17,29.12 17.13,29.25 17.13,29.28 Y2.P$3 19.2,31.35 C21.1
N$13
  Top 0.152: U1.24 12.6,28.32 C20.2 15,30.95 Y2.P$1
N$14
  Top 0.152: D3.2 0.82,20.9 R13.1
N$15
  Top 0.152: R12.1 0.82,21.9 D2.2
N$16
  Top 0.152: D4.2 2.83,19.85 R16.1
N$17
  Top 0.152: R19.2 R18.2 R17.1
N$18
  Top 0.152: U4.13 27.48,28.5 R14.2
N$19
  Top 0.152: U4.14 27.52,29.15 R15.2
OA1
  Top 0.813: U3.6 8.87,8.36 8.34,7.83 8.34,5.57 8.67,5.24 13.33,5.24 J3.1
OA2
  Top 0.813: U3.8 11.4,8.59 12.16,7.83 12.16,7.4 12.85,6.71 15.44,6.71 18.14,4 J3.2
OB1
  Top 0.813: J3.3 21.95,4 24.66,6.71 27.4,6.71 27.84,7.15 27.84,7.83 28.66,8.65 U2.6
OB2
  Top 0.813: U2.8 31.2,8.29 31.66,7.83 31.66,5.57 31.33,5.24 26.67,5.24 J3.4
RE  (via drill 0.3)
  Top 0.152: U4.2 19.44,28.5 v19,28.94 | U1.28 10.31,28.99 10.31,30.02 10.02,30.31 10.02,30.91 9.89,31.05 9.52,31.05 v9.2,31.36
  Route2 0.152: v19,28.94 18.4,29.54 18.4,29.98 17.88,30.5 14.7,30.5 14.14,31.05 13.66,31.05 13.32,30.71 13.32,30.57 13,30.26 12.88,30.26 11.83,29.2 9.97,29.2 9.48,29.2 9.14,29.54 9.14,30.02 9.2,30.08 v9.2,31.36
RESET  (via drill 0.3)
  Top 0.152: S1.P$4 23.48,33.02 R3.2 C1.1 20.48,33.02 17.1,36.4 17.1,37.74 J2.10 16.39,36.69 v16.3,36.6 | v4.64,26.38 4.96,26.7 U1.40
  Route2 0.152: v16.3,36.6 14.5,34.8 10,34.8 5.8,30.6 5,30.6 3.7,29.3 3.7,27.32 v4.64,26.38
SWDCLK  (via drill 0.3)
  Top 0.152: U1.45 4.78,24.2 v4.76,24.22 4.37,24.22 4.22,24.07 3.51,24.07 3.34,23.9 3.34,23.45 2.83,22.94 R4.2 | J2.4 12.58,36.78 v12.4,36.6
  Route2 0.152: v12.4,36.6 10.9,35.1 9.87,35.1 5.67,30.91 4.87,30.91 3.36,29.39 3.36,25.62 v4.76,24.22
SWDIO  (via drill 0.3)
  Top 0.152: U1.46 5.47,23.57 5.16,23.57 5.07,23.48 v4.2,23.48 | v11.1,36.6 11.31,36.81 J2.2
  Route2 0.152: v4.2,23.48 4.1,23.59 4.1,24.39 3.05,25.43 3.05,29.52 4.75,31.21 5.55,31.21 9.75,35.41 9.91,35.41 v11.1,36.6
TERM  (via drill 0.3)
  Top 0.152: U4.5 v19.11,26.55 v19.1,26.54 | v13.9,30.47 13.69,30.26 12.88,30.26 12.23,29.6 11.6,29.6 11.35,29.35 U1.26
  Route2 0.152: v19.1,26.54 19.1,28.3 19.04,28.36 18.76,28.36 18.42,28.7 18.42,29.09 18.09,29.41 18.09,29.85 17.75,30.19 14.18,30.19 v13.9,30.47
USBDM  (via drill 0.3)
  Top 0.152: v26.06,33.6 26.06,33.8 25.85,34.01 X1.D- | U1.33 7.82,28.98 7.82,29.3 7.62,29.49 v7.62,29.91
  Route2 0.152: v7.62,29.91 7.62,30.79 10.13,33.3 24.68,33.3 24.96,33.02 25.48,33.02 v26.06,33.6
USBDP  (via drill 0.3)
  Top 0.152: X1.D+ v25.2,33.6 | U1.34 7.32,28.98 7.32,29.3 6.71,29.9 v6.7,29.9
  Route2 0.152: v25.2,33.6 10,33.6 6.7,30.3 v6.7,29.9
VDDCORE
  Top 0.152: C2.1 2,25.2 L1.2 | C2.1 3.05,27.15 C3.1 | U1.41 5.47,26.07 5.16,26.07 4.89,25.8 4.4,25.8 C2.1
VSENSE  (via drill 0.3)
  Top 0.152: v10.4,18.62 10.35,18.67 U1.9 | R19.1 4.03,16.48 v3.9,16.6
  Route2 0.152: v10.4,18.62 9.48,17.7 4.8,17.7 3.9,16.8 v3.9,16.6
VSW
  Top 0.152: L1.1 U1.43
Y  (via drill 0.3)
  Top 0.152: U4.10 v27.45,26.55 v27.46,26.54 | v28.5,25.5 29.69,24.31 J1.7
  Route2 0.152: v27.46,26.54 v28.5,25.5
Z  (via drill 0.3)
  Top 0.152: U4.12 26.18,27.75 27.26,27.75 27.29,27.72 27.49,27.72 v28.07,27.14 | v29.11,26.11 30.18,25.04 34.21,25.04 34.94,24.31 J1.8
  Route2 0.152: v28.07,27.14 | v28.07,27.14 v29.11,26.11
